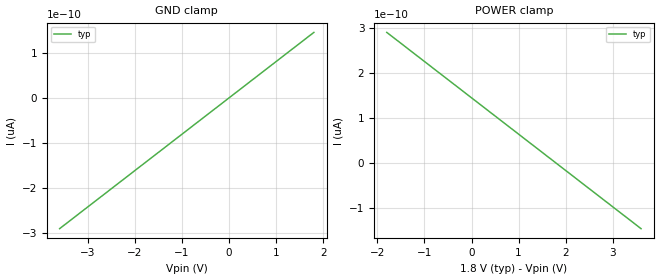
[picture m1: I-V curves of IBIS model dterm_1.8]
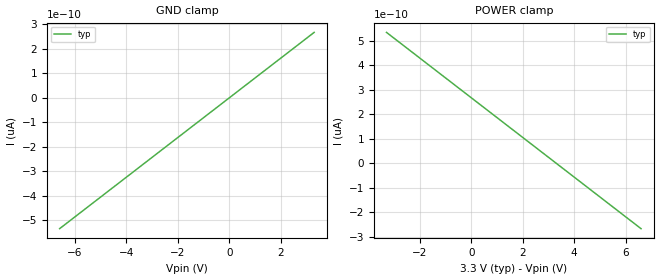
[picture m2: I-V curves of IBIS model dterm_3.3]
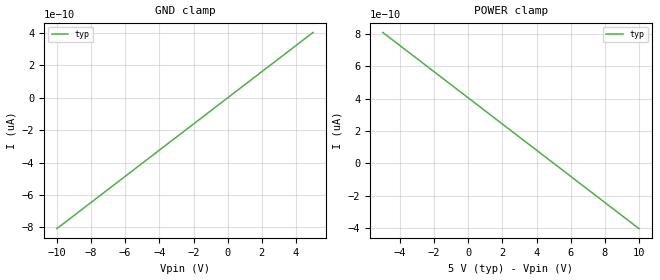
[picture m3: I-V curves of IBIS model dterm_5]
|Texas Instruments Incorporated
|tmux1574, 4 Data Lane 2:1 5V Precision mux
[IBIS Ver]   4.1
[File name]   tmux1574.ibs
[Date]   07/14/22
[File Rev]   1.0
[Source]
| Texas Instruments Incorporated.
| ASC-INT-MPD
| 12500 TI Blvd
| Dallas, TX - 75243
[Notes]   Revision History:
| Rev 1.0: 07/14/22
| - Initial version of the model
| - Model generated from simulations in SPECTRE
| - C_comp although listed in numerical order of value are
|   obtained from varying PVT conditions. For PVT conditions for
|   each specific value refer the buffer description under
|   respective [Model]. IBIS model user is responsible for using
|   appropriate C_comp to simulate for Signal Integrity.
[Disclaimer]
| This model is designed as an aid for customers of Texas Instruments.
| TI and its licensors and suppliers make no warranties, either expressed
| or implied, with respect to this  model, including the warranties of
| merchantability or fitness for a particular purpose. The model is
| provided solely on an "as is" basis. The entire risk as to its quality
| and performance is with the customer.
| This model is subject to change without notice. Texas Instruments
| Incorporated is not responsible for updating this model.
[Copyright]
(C) Copyright 2022 Texas Instruments Incorporated.All rights reserved.
|  Component TMUX1574PW 16-pin - PW package
|  Part # TMUX1574PW
[Component]   TMUX1574PW
[Manufacturer]  TI
[Package]
|   typ   min   max
R_pkg   0.0668   NA   NA
L_pkg   2.1992nH   NA   NA
C_pkg   0.2884pF   NA   NA
[Pin]   signal_name   model_name
   1   SEL   inbuf
   2   S1A   sterm
   3   S1B   sterm
   4   D1   dterm
   5   S2A   sterm
   6   S2B   sterm
   7   D2   dterm
   8   GND   gnd
   9   D3   dterm
   10   S3B   sterm
   11   S3A   sterm
   12   D4   dterm
   13   S4B   sterm
   14   S4A   sterm
   15   ENZ   inbuf
   16   VDD   power
[Series Switch Groups]
On 1 /
On 2 /
Off 1 2 /
[Series Pin Mapping]  pin_2 model_name function_table_group
   2   4   switch_1.8   1
   5   7   switch_1.8   1
  11   9   switch_1.8   1
  14  12   switch_1.8   1
   3   4   switch_1.8   2
   6   7   switch_1.8   2
  10   9   switch_1.8   2
  13  12   switch_1.8   2
|   2   4   switch_3.3   1
|   5   7   switch_3.3   1
|  11   9   switch_3.3   1
|  14  12   switch_3.3   1
|   3   4   switch_3.3   2
|   6   7   switch_3.3   2
|  10   9   switch_3.3   2
|  13  12   switch_3.3   2
|   2   4   switch_5   1
|   5   7   switch_5   1
|  11   9   switch_5   1
|  14  12   switch_5   1
|   3   4   switch_5   2
|   6   7   switch_5   2
|  10   9   switch_5   2
|  13  12   switch_5   2
|  Component TMUX1574DYY 16-pin - DYY package
|  Part # TMUX1574DYY
[Component]   TMUX1574DYY
[Manufacturer]  TI
[Package]
|   typ   min   max
R_pkg   0.0668   NA   NA
L_pkg   2.1992nH   NA   NA
C_pkg   0.2884pF   NA   NA
[Pin]   signal_name   model_name
   1   SEL   inbuf
   2   S1A   sterm
   3   S1B   sterm
   4   D1   dterm
   5   S2A   sterm
   6   S2B   sterm
   7   D2   dterm
   8   GND   gnd
   9   D3   dterm
   10   S3B   sterm
   11   S3A   sterm
   12   D4   dterm
   13   S4B   sterm
   14   S4A   sterm
   15   ENZ   inbuf
   16   VDD   power
[Series Switch Groups]
On 1 /
On 2 /
Off 1 2 /
[Series Pin Mapping]  pin_2 model_name function_table_group
   2   4   switch_1.8   1
   5   7   switch_1.8   1
  11   9   switch_1.8   1
  14  12   switch_1.8   1
   3   4   switch_1.8   2
   6   7   switch_1.8   2
  10   9   switch_1.8   2
  13  12   switch_1.8   2
|   2   4   switch_3.3   1
|   5   7   switch_3.3   1
|  11   9   switch_3.3   1
|  14  12   switch_3.3   1
|   3   4   switch_3.3   2
|   6   7   switch_3.3   2
|  10   9   switch_3.3   2
|  13  12   switch_3.3   2
|   2   4   switch_5   1
|   5   7   switch_5   1
|  11   9   switch_5   1
|  14  12   switch_5   1
|   3   4   switch_5   2
|   6   7   switch_5   2
|  10   9   switch_5   2
|  13  12   switch_5   2
|  Component TMUX1574RSV 16-pin - RSV package
|  Part # TMUX1574RSV
[Component]   TMUX1574RSV
[Manufacturer]  TI
[Package]
|   typ   min   max
R_pkg   0.0668   NA   NA
L_pkg   2.1992nH   NA   NA
C_pkg   0.2884pF   NA   NA
[Pin]   signal_name   model_name
   1   S1B   sterm
   2   D1   dterm
   3   S2A   sterm
   4   S2B   sterm
   5   D2   dterm
   6   GND   gnd
   7   D3   dterm
   8   S3B   sterm
   9   S3A   sterm
   10   D4   dterm
   11   S4B   sterm
   12   S4A   sterm
   13   ENZ   inbuf
   14   VDD   power
   15   SEL   inbuf
   16   S1A   sterm
[Series Switch Groups]
On 1 /
On 2 /
Off 1 2 /
[Series Pin Mapping]  pin_2 model_name function_table_group
  16   2   switch_1.8   1
   3   5   switch_1.8   1
   9   7   switch_1.8   1
  12  10   switch_1.8   1
   1   2   switch_1.8   2
   4   5   switch_1.8   2
   8   7   switch_1.8   2
  11  10   switch_1.8   2
|  16   2   switch_3.3   1
|   3   5   switch_3.3   1
|   9   7   switch_3.3   1
|  12  10   switch_3.3   1
|   1   2   switch_3.3   2
|   4   5   switch_3.3   2
|   8   7   switch_3.3   2
|  11  10   switch_3.3   2
|  16   2   switch_5   1
|   3   5   switch_5   1
|   9   7   switch_5   1
|  12  10   switch_5   1
|   1   2   switch_5   2
|   4   5   switch_5   2
|   8   7   switch_5   2
|  11  10   switch_5   2
[Model Selector] dterm
dterm_1.8 Use for operation at 1V
dterm_3.3 Use for operation at 3V
dterm_5 Use for operation at 5V
[Model Selector] sterm
sterm_1.8 Use for operation at 1V
sterm_3.3 Use for operation at 3V
sterm_5 Use for operation at 5V
[Model Selector] inbuf
inbuf_1.8 Use for operation at 1V
inbuf_3.3 Use for operation at 3V
inbuf_5 Use for operation at 5V
| switch_1.8
[Model]   switch_1.8
Model_type   Series_switch
|   typ   min   max
C_comp   4.014581e-12   NA   NA
[Voltage Range]   1.8   NA   NA
[Power Clamp Reference]   1.8   NA   NA
[Temperature Range]   27   NA   NA
[On]
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[Off]
|   typ   min   max
[R Series]   10G   NA   NA
| switch_3.3
[Model]   switch_3.3
Model_type   Series_switch
|   typ   min   max
C_comp   4.014581e-12   NA   NA
[Voltage Range]   3.3   NA   NA
[Power Clamp Reference]   3.3   NA   NA
[Temperature Range]   27   NA   NA
[On]
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[Off]
|   typ   min   max
[R Series]   10G   NA   NA
| switch_5
[Model]   switch_5
Model_type   Series_switch
|   typ   min   max
C_comp   4.014581e-12   NA   NA
[Voltage Range]   5   NA   NA
[Power Clamp Reference]   5   NA   NA
[Temperature Range]   27   NA   NA
[On]
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[Off]
|   typ   min   max
[R Series]   10G   NA   NA
| Models and submodels in the file (12): dterm_1.8 (Terminator), dterm_3.3 (Terminator), dterm_5 (Terminator), switch_1.8 (Series_switch), switch_3.3 (Series_switch), switch_5 (Series_switch), sterm_1.8 (Terminator), sterm_3.3 (Terminator), sterm_5 (Terminator), inbuf_1.8 (Input), inbuf_3.3 (Input), inbuf_5 (Input)
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| dterm_1.8
[Model]   dterm_1.8
Model_type   Terminator
|   typ   min   max
C_comp   4.014581e-12   NA   NA
[Voltage Range]   1.8   NA   NA
[Temperature Range]   27   NA   NA
[Power Clamp Reference]   1.8   NA   NA
[GND Clamp Reference]   0   NA   NA
[GND Clamp]
|   Voltage   I(typ)   I(min)   I(max)
-3.6V     0A         NA         NA
-1.636V   0A         NA         NA
545.5mV   0A         NA         NA
1.8V      0A         NA         NA
[POWER Clamp]
|   Voltage   I(typ)   I(min)   I(max)
-1.8V     0A         NA         NA
1.2V      0A         NA         NA
3.055V    0A         NA         NA
3.6V      0A         NA         NA
| dterm_3.3
[Model]   dterm_3.3
Model_type   Terminator
|   typ   min   max
C_comp   4.014581e-12   NA   NA
[Voltage Range]   3.3   NA   NA
[Temperature Range]   27   NA   NA
[Power Clamp Reference]   3.3   NA   NA
[GND Clamp Reference]   0   NA   NA
[GND Clamp]
|   Voltage   I(typ)   I(min)   I(max)
-6.6V     0A         NA         NA
-6.4V     0A         NA         NA
200mV     0A         NA         NA
3.3V      0A         NA         NA
[POWER Clamp]
|   Voltage   I(typ)   I(min)   I(max)
-3.3V     0A         NA         NA
1.3V      0A         NA         NA
3.1V      0A         NA         NA
6.6V      0A         NA         NA
| dterm_5
[Model]   dterm_5
Model_type   Terminator
|   typ   min   max
C_comp   4.014581e-12   NA   NA
[Voltage Range]   5   NA   NA
[Temperature Range]   27   NA   NA
[Power Clamp Reference]   5   NA   NA
[GND Clamp Reference]   0   NA   NA
[GND Clamp]
|   Voltage   I(typ)   I(min)   I(max)
-10V      0A         NA         NA
454.5mV   0A         NA         NA
606.1mV   0A         NA         NA
5V        0A         NA         NA
[POWER Clamp]
|   Voltage   I(typ)   I(min)   I(max)
-5V       0A         NA         NA
-4.091V   0A         NA         NA
-3.333V   0A         NA         NA
10V       0A         NA         NA
